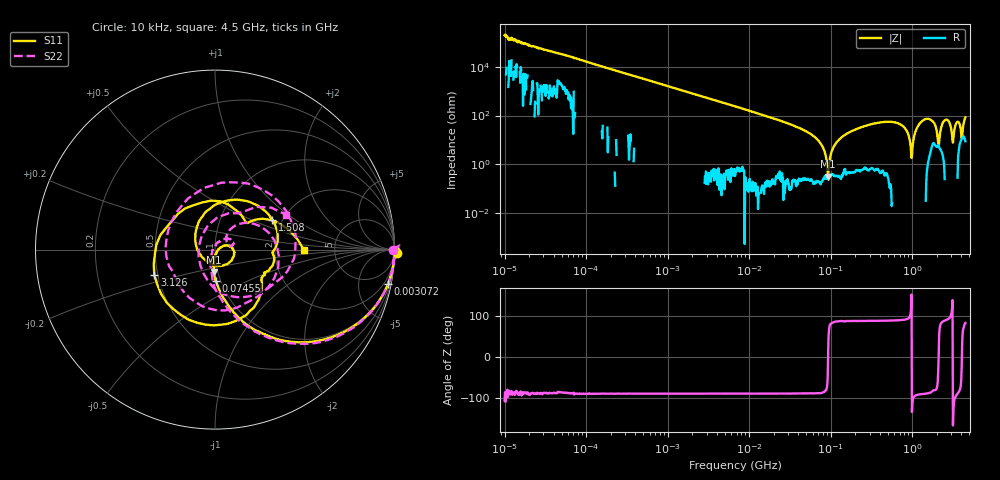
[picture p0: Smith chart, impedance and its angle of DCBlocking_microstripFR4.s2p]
!Siglent Technologies,SNA5004A,SNA5XCED5R0097,V1.0.0.2.10.R9
!Date: 2024-10-18 16:04:56
!Data & Calibration Information:
!Freq	S11:F2(ON)	S21:F2(ON)	S12:F2(ON)	S22:F2(ON)
# Hz S DB R 50
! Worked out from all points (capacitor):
!   1001 points, 10 kHz to 4.5 GHz, reference 50 ohm
!   read as one part in series: C = 101 pF near 10.67 kHz
!   lowest |Z| = 313 mohm at 93.02 MHz (marker M1)
!   series resonance near 93.09 MHz, so ESL is about 29 nH
!   S11 on the Smith chart (normalised r, x): 10 kHz: -62, -71; 3.072 MHz: 1, -10; 74.55 MHz: 0.95, -0.34; 1.508 GHz: 1.77, +0.68; 3.126 GHz: 0.48, -0.16; 4.5 GHz: 2.96, -0.00
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10000  0.12 -0.9  -65.77 106.0  -65.62 87.5  -0.10 -0.2
87919.76  -0.03 -0.4  -45.37 90.5  -45.36 89.9  -0.07 -0.5
772988.4  -0.00 -2.9  -26.37 87.1  -26.31 87.1  -0.01 -3.0
3071945  -0.15 -11.3  -14.47 78.6  -14.46 78.6  -0.17 -11.4
6708204  -0.71 -23.6  -8.27 66.1  -8.25 66.2  -0.71 -24.0
1.827695e7  -3.70 -51.5  -2.44 37.9  -2.44 37.9  -3.71 -52.5
5.897837e7  -12.57 -82.9  -0.27 4.4  -0.28 4.4  -12.62 -87.9
7.45505e7  -15.26 -88.8  -0.16 -1.4  -0.16 -1.4  -15.18 -94.0
9.301547e7  -18.03 -92.7  -0.10 -7.2  -0.11 -7.2  -18.12 -100.0
1.903189e8  -36.30 -15.2  -0.06 -29.5  -0.08 -29.5  -39.05 138.9
2.740134e8  -24.74 22.1  -0.12 -45.8  -0.13 -45.8  -24.95 57.9
5.185364e8  -19.31 -25.1  -0.23 -90.1  -0.24 -90.1  -19.35 21.4
7.369126e8  -21.67 -99.5  -0.26 -129.1  -0.27 -129.0  -21.80 17.8
9.941224e8  -16.69 137.3  -0.39 -175.5  -0.40 -175.4  -16.70 52.6
1.507796e9  -8.87 27.7  -1.10 94.8  -1.11 94.8  -8.75 -15.0
1.785807e9  -9.92 -3.1  -1.50 47.5  -1.50 47.5  -9.29 -63.9
2.115077e9  -10.11 -27.1  -1.18 -7.9  -1.18 -7.9  -11.31 -160.2
2.571132e9  -8.12 -60.3  -1.51 -89.8  -1.50 -89.8  -7.72 63.4
3.125522e9  -8.72 -157.4  -1.81 176.9  -1.79 177.0  -7.76 -21.0
3.701812e9  -11.62 73.9  -1.42 77.4  -1.41 77.4  -12.52 -85.1
4.054962e9  -12.51 39.1  -1.26 11.7  -1.25 11.7  -19.46 133.9
4.5e9  -6.11 -0.1  -2.27 -68.7  -2.30 -68.7  -7.12 26.2
